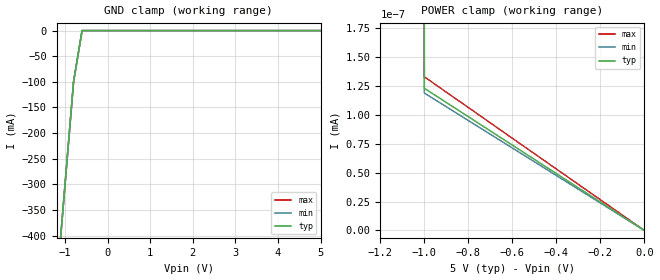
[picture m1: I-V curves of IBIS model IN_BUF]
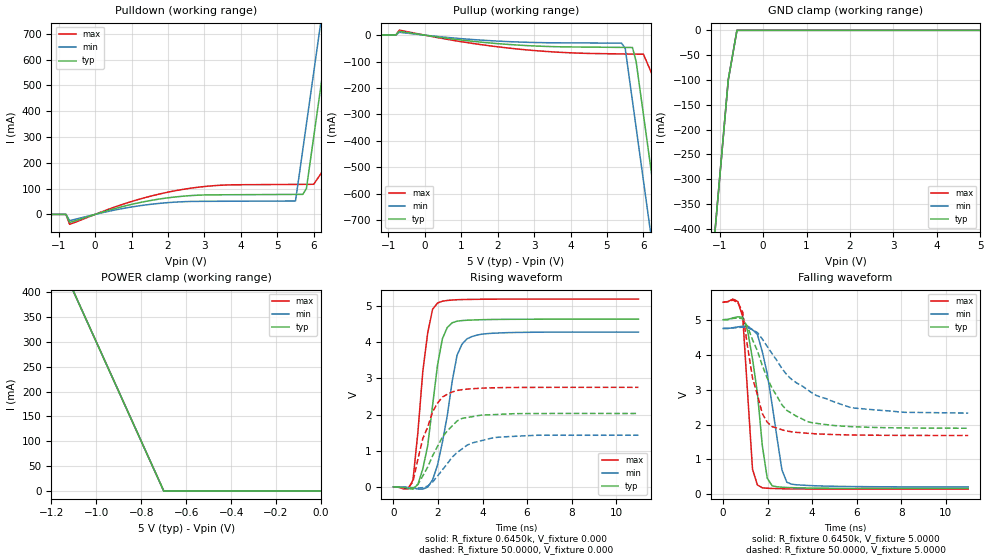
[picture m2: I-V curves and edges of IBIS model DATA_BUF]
| IBIS file m48t35_pdip28.ibs created by s2ibis2 version 1.1
| North Carolina State University Electronics Research Laboratory  1995
[IBIS ver]   2.1
[File name]   m48t35_pdip28.ibs
[File Rev]   4.0
[Date]   September 12, 2002
[Source]   ST models
[Notes]   Extracted view used. Simulation with Eldo (the s2ibis2 code
   was slightly changed to run with Eldo)
[Disclaimer] We used the packaging information of the T212. It should be
   the same but need to be confirme. We also put a 1.0 ohm
   resistor in series with the output and input for current
   limitation.
[Copyright]   ST Microelectronics Inc.
|   Component m48t35
[Component]   m48t35
[Manufacturer]   ST Microelectronics [Package]
[Package]
| variable   typ   min   max
R_pkg   2.0000m   2.0000m   2.0000m
L_pkg   9.5000nH   4.2000nH   14.8000nH
C_pkg   2.1000pF   1.4000pF   2.9000pF
[Pin]  signal_name   model_name   R_pin   L_pin   C_pin
| gdb  dummy   dummy
| od   dummy   dummy
| pd   dummy   dummy
1   A14   IN_BUF
2   A12   IN_BUF
3   A7   IN_BUF
4   A6   IN_BUF
5   A5   IN_BUF
6   A4   IN_BUF
7   A3   IN_BUF
8   A2   IN_BUF
9   A1   IN_BUF
10   A0   IN_BUF
11   DQ0   DATA_BUF
12   DQ1   DATA_BUF
13   DQ2   DATA_BUF
14   VSS   GND
15   DQ3   DATA_BUF
16   DQ4   DATA_BUF
17   DQ5   DATA_BUF
18   DQ6   DATA_BUF
19   DQ7   DATA_BUF
20   E#   IN_BUF
21   A10   IN_BUF
22   G#   IN_BUF
23   A11   IN_BUF
24   A9   IN_BUF
25   A8   IN_BUF
26   A13   IN_BUF
27   W#   IN_BUF
28   VCC   POWER
| Models and submodels in the file (2): IN_BUF (Input), DATA_BUF (I/O)
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|   Model IN_BUF
[Model]   IN_BUF
Model_type   Input
Vinl =   0.8000V
Vinh =   2.2000V
C_comp   2.0100pF   1.9700pF   2.0600pF
[Temperature Range]   27.0000   70.0000   0.000
[Voltage Range]   5.0000V   4.7500V   5.5000V
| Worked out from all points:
|   GND clamp passes 1 mA (typ) near -0.60 V on its own axis
|   POWER clamp passes 1 mA (typ) near -1.32 V on its own axis
[GND_clamp]
| voltage   I(typ)   I(min)   I(max)
-5V       -4.3A      -4.3A      -4.3A
-1.2V     -500mA     -500mA     -500mA
-1V       -300mA     -300mA     -300mA
-800mV    -100mA     -100mA     -100mA
-600mV    -2.424uA   -939.7nA   -1.758uA
5V        2.595nA    12.35pA    3.525nA
[POWER_clamp]
| voltage   I(typ)   I(min)   I(max)
-5V       3.437A     3.385A     3.471A
-1.1V     57.92nA    90.84nA    42.02nA
-1V       123.1pA    119pA      133.1pA
0V        0A         0A         0A
|   Model DATA_BUF
[Model]   DATA_BUF
Model_type   I/O
Polarity   Inverting
Enable   Active-High
Vinl =   0.8000V
Vinh =   2.2000V
Vmeas =   1.5000V
Cref =1.000e-10F
Rref =   0.6420k
Vref =   1.7500V
C_comp   4.3700pF   4.2600pF   4.4800pF
[Temperature Range]   27.0000   70.0000   0.000
[Voltage Range]   5.0000V   4.7500V   5.5000V
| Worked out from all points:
|   slope of the pulldown table from 0 to 0.75 V, typ, clamps not added: 24.6 ohm
|   slope of the pullup table from 0 to 0.75 V, typ, clamps not added: 52.7 ohm
|   GND clamp passes 1 mA (typ) near -0.60 V on its own axis
|   POWER clamp passes 1 mA (typ) near -0.70 V on its own axis
|   rising waveform, R_fixture 0.6450k, V_fixture 0.000: 20-80 % time 616ps typ, 724ps min, 497ps max; typ from 0 V to 4.64 V
|   rising waveform, R_fixture 50.0000, V_fixture 0.000: 20-80 % time 1.13ns typ, 1.32ns min, 852ps max; typ from 0 V to 2.03 V
|   falling waveform, R_fixture 0.6450k, V_fixture 5.0000: 20-80 % time 543ps typ, 695ps min, 323ps max; typ from 5 V to 0.169 V
|   falling waveform, R_fixture 50.0000, V_fixture 5.0000: 20-80 % time 1.36ns typ, 2.32ns min, 719ps max; typ from 5 V to 1.89 V
[Pulldown]
| voltage   I(typ)   I(min)   I(max)
-5V       0A         0A         0A
-800mV    0A         0A         0A
-700mV    -31.52mA   -24.2mA    -38.45mA
2.3V      69.1mA     48.42mA    94.27mA
5.5V      77.53mA    52.02mA    116.3mA
5.7V      77.69mA    250mA      116.5mA
5.8V      100mA      350mA      116.6mA
6V        300mA      550mA      116.8mA
6.4V      700mA      950mA      200mA
6.8V      1.1A       1.35A      600mA
7.2V      1.5A       1.75A      1A
10V       4.3A       4.55A      3.8A
[Pullup]
| voltage   I(typ)   I(min)   I(max)
-5V       0A         0A         0A
-700mV    14.66mA    10.82mA    18.98mA
2.4V      -36.11mA   -25.03mA   -50.31mA
5.4V      -46.31mA   -30.2mA    -71.02mA
5.5V      -46.43mA   -50mA      -71.22mA
5.7V      -46.79mA   -250mA     -71.62mA
5.8V      -100mA     -350mA     -71.82mA
6V        -300mA     -550mA     -72.21mA
6.4V      -700mA     -950mA     -200mA
6.8V      -1.1A      -1.35A     -600mA
7.2V      -1.5A      -1.75A     -1A
10V       -4.3A      -4.55A     -3.8A
[GND_clamp]
| voltage   I(typ)   I(min)   I(max)
-5V       -4.3A      -4.3A      -4.3A
-1.2V     -500mA     -500mA     -500mA
-1V       -300mA     -300mA     -300mA
-800mV    -100mA     -100mA     -100mA
-600mV    -26.04uA   -10.29uA   -17.63uA
5V        60.14pA    9.461nA    9.57nA
[POWER_clamp]
| voltage   I(typ)   I(min)   I(max)
-5V       4.3A       4.3A       4.3A
-1.1V     400mA      400mA      400mA
-1V       300mA      300mA      300mA
-700mV    12.45uA    2.467uA    49.04uA
0V        0A         0A         0A
[Ramp]
| variable   typ   min   max
dV/dt_r   2.7824/0.5727n   2.5686/0.7949n   3.1163/0.4338n
dV/dt_f   2.8983/0.4602n   2.7219/0.6943n   3.2101/0.3288n
R_load = 0.6420k
[Rising Waveform]
R_fixture = 0.6450k
V_fixture = 0.000
V_fixture_min = 0.000
V_fixture_max = 0.000
| time   V(typ)   V(min)   V(max)
0s        1.338nV    1.705nV    1.151nV
880ps     -64.36mV   -32.79mV   190.4mV
1.32ns    493.9mV    -64.4mV    3.19V
1.54ns    1.137V     -6.774mV   4.257V
1.76ns    2.255V     192.7mV    4.914V
1.98ns    3.364V     600.1mV    5.085V
2.42ns    4.411V     1.974V     5.157V
2.86ns    4.584V     3.644V     5.177V
3.3ns     4.609V     4.094V     5.185V
11ns      4.639V     4.283V     5.195V
[Rising Waveform]
R_fixture = 50.0000
V_fixture = 0.000
V_fixture_min = 0.000
V_fixture_max = 0.000
| time   V(typ)   V(min)   V(max)
0s        961.2pV    1.127nV    873.9pV
660ps     -33.19mV   -13.8mV    -34.1mV
880ps     -38.76mV   -22.34mV   143mV
1.32ns    300.7mV    -22.88mV   1.334V
1.76ns    857.6mV    132.2mV    2.076V
2.2ns     1.377V     469.8mV    2.484V
2.64ns    1.686V     822.4mV    2.624V
3.52ns    1.939V     1.212V     2.713V
4.62ns    2.001V     1.368V     2.742V
11ns      2.03V      1.429V     2.753V
[Falling Waveform]
R_fixture = 0.6450k
V_fixture = 5.0000
V_fixture_min = 4.7500
V_fixture_max = 5.5000
| time   V(typ)   V(min)   V(max)
0s        5V         4.75V      5.5V
660ps     5.084V     4.793V     5.521V
880ps     5.07V      4.814V     5.085V
1.32ns    3.88V      4.712V     717.5mV
1.54ns    2.899V     4.578V     269mV
1.76ns    1.392V     4.081V     187.8mV
1.98ns    465.1mV    3.458V     175.2mV
2.64ns    204.9mV    700.5mV    161.6mV
2.86ns    197mV      347.5mV    159.1mV
11ns      168.7mV    212.6mV    149.1mV
[Falling Waveform]
R_fixture = 50.0000
V_fixture = 5.0000
V_fixture_min = 4.7500
V_fixture_max = 5.5000
| time   V(typ)   V(min)   V(max)
0s        5V         4.75V      5.5V
660ps     5.05V      4.777V     5.494V
880ps     5.029V     4.786V     5.211V
1.32ns    4.424V     4.711V     3.33V
1.76ns    3.685V     4.447V     2.311V
2.2ns     3.038V     4.028V     1.939V
2.86ns    2.404V     3.423V     1.813V
3.74ns    2.092V     3.016V     1.751V
5.72ns    1.94V      2.488V     1.701V
11ns      1.893V     2.327V     1.686V
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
